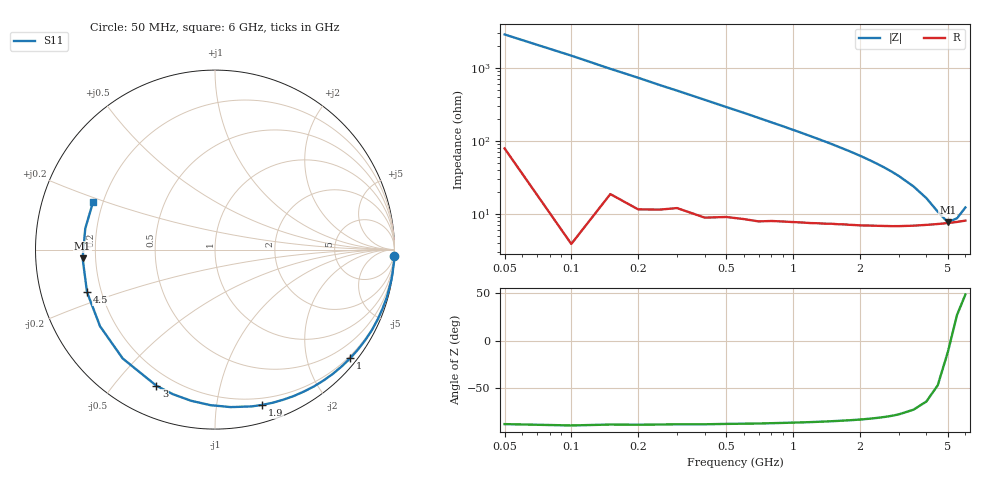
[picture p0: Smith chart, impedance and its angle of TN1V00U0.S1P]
! SIEMENS Discrete & RF Semiconductors
! BAS70-07W
! Si Schottky Diode in SOT343
! VR = 1 V
! S-Parameters:  February  1997
# GHz  S  MA  R  50
!  f  S11
! GHz  MAG  ANG
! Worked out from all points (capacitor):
!   34 points, 50 MHz to 6 GHz, reference 50 ohm
!   read as one part to ground: C = 1.09 pF near 50 MHz
!   lowest |Z| = 7.68 ohm at 5 GHz (marker M1)
!   series resonance near 5.145 GHz, so ESL is about 880 pH
!   S11 on the Smith chart (normalised r, x): 50 MHz: 2, -57; 1 GHz: 0.15, -2.83; 1.9 GHz: 0.14, -1.34; 3 GHz: 0.14, -0.65; 4.5 GHz: 0.15, -0.16; 6 GHz: 0.16, +0.18
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0.05  0.999 -2.0
0.1  0.9998 -3.9
0.2  0.9979 -7.8
0.4  0.9935 -15.6
0.6  0.9862 -23.3
0.7  0.9826 -27.2
0.8  0.9772 -31.1
0.9  0.972 -34.9
1  0.9663 -38.8
1.1  0.9604 -42.6
1.2  0.9542 -46.5
1.3  0.9474 -50.3
1.4  0.9407 -54.1
1.6  0.9263 -61.8
1.8  0.9118 -69.3
1.9  0.9043 -73.1
2  0.8974 -76.8
2.2  0.8819 -84.3
2.4  0.867 -91.7
2.6  0.8527 -99.0
2.8  0.8391 -106.2
3  0.8258 -113.3
3.5  0.7952 -130.3
4  0.7699 -146.3
4.5  0.7514 -161.6
5  0.7392 -176.2
5.5  0.7323 170.7
6  0.7292 158.6
